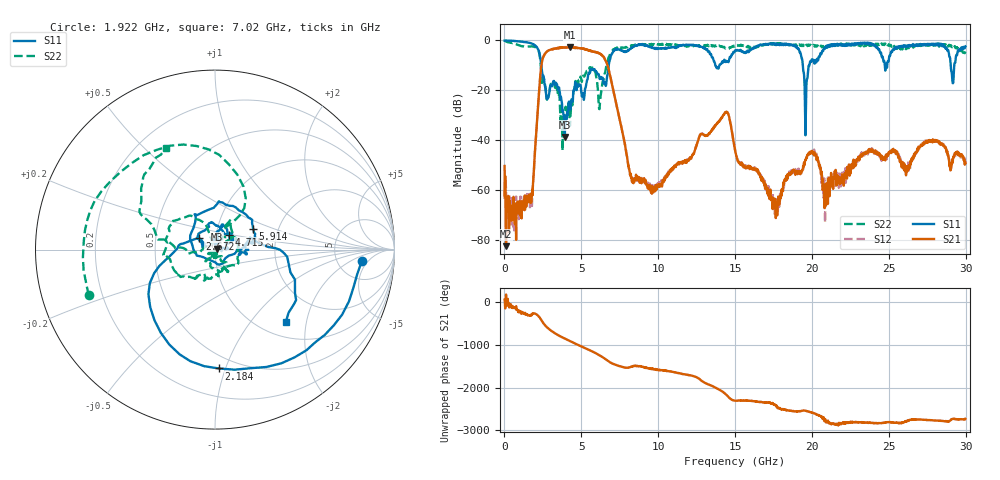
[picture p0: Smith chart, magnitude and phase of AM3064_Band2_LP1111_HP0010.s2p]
# Hz S DB R 50.0
!freq dBS11 angS11 dBS21 angS21 dBS12 angS12 dBS22 angS22
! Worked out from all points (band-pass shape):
!   1600 points, 10 MHz to 29.98 GHz, reference 50 ohm
!   highest |S21| = -2.74 dB at 4.246 GHz (marker M1); lowest = -82.5 dB at 103.7 MHz (marker M2)
!   |S21| within 3 dB of the highest: 2.596 GHz to 6.302 GHz (3.706 GHz wide, 83.3 % of centre)
!   lowest |S11| = -38.7 dB at 3.927 GHz (marker M3), VSWR 1.02, Z = 51.1 + j0.424 ohm
!   |S11| at or under -10 dB: 2.394 GHz to 6.785 GHz (4.391 GHz wide, 95.7 % of centre); 13.71 GHz to 13.98 GHz (263 MHz wide, 1.9 % of centre); 19.41 GHz to 19.83 GHz (426.6 MHz wide, 2.17 % of centre)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
!   |S22| runs from -44.2 to -0.1 dB; largest |S21 - S12| = 0.021
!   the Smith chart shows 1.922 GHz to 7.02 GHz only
!   S11 on the Smith chart (normalised r, x): 1.922 GHz: 8.74, -3.45; 2.184 GHz: 0.40, -0.95; 2.672 GHz: 0.83, +0.11; 4.715 GHz: 1.15, +0.19; 5.914 GHz: 1.49, +0.37; 7.02 GHz: 1.29, -1.52
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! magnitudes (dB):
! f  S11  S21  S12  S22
! 10 MHz  -0.1  -50.3  -60.1  -0.1
! 103.7 MHz  0.0  -82.5  -59.6  -0.4
! 1.153 GHz  -0.6  -67.2  -67.1  -2.3
! 1.922 GHz  -1.7  -50.9  -51.6  -2.5
! 2.184 GHz  -3.6  -26.3  -26.2  -3.8
! 2.672 GHz  -19.4  -5.1  -5.0  -18.9
! 3.927 GHz  -38.7  -2.8  -2.7  -30.3
! 4.246 GHz  -25.1  -2.7  -2.8  -33.5
! 4.715 GHz  -18.9  -3.0  -2.9  -17.6
! 5.015 GHz  -21.5  -3.2  -3.1  -16.0
! 5.914 GHz  -12.3  -4.7  -4.6  -12.8
! 7.02 GHz  -5.0  -18.2  -18.1  -4.0
! 8.276 GHz  -2.8  -55.2  -54.7  -2.1
! 10 GHz  -3.3  -57.7  -57.2  -1.6
! 14.37 GHz  -8.6  -28.8  -28.7  -3.2
! 15 GHz  -4.0  -44.2  -44.2  -2.1
! 17.67 GHz  -1.9  -66.9  -70.2  -1.4
! 19.58 GHz  -38.0  -47.8  -48.5  -2.1
! 19.99 GHz  -7.6  -44.6  -44.7  -1.7
! 20.87 GHz  -2.8  -58.0  -61.6  -2.7
! 25 GHz  -8.0  -44.7  -45.0  -1.6
! 29.98 GHz  -2.4  -49.3  -48.8  -4.4
